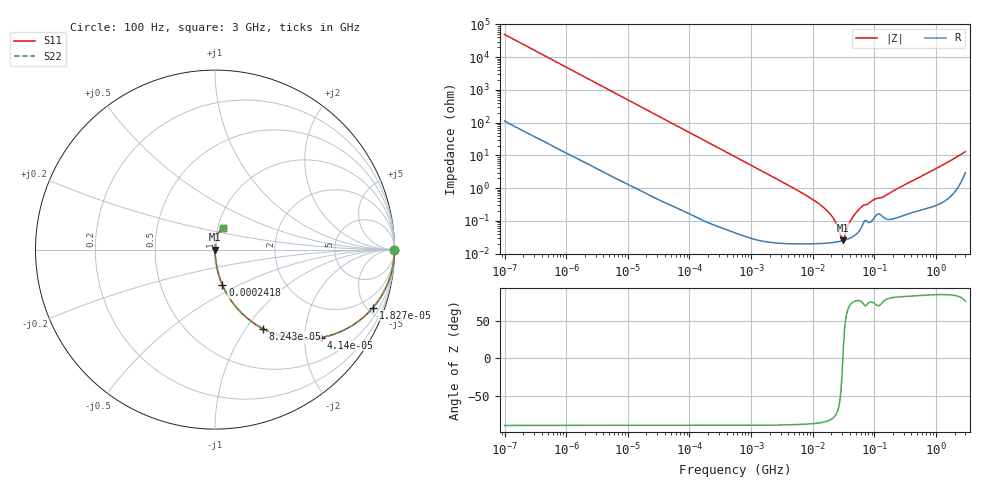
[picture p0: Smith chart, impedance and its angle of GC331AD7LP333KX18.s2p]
!Murata Part Number: GC331AD7LP333KX18
!These Parameters are Measured in Series Mode Connection
!Data Generated on Jun 10, 2025
!  o--ll--o
!Port1  Port2
!  o------o
!Operation Temp=25[degC], DC Bias Voltage=0[V]
!Freq. Start=100[Hz] Stop=3[GHz] 401[Steps]
# Hz S RI R 50
!Freq.(Hz) S11(Real) S11(Imag) S21(Real) S21(Imag) S12(Real) S12(Imag) S22(Real) S22(Imag)
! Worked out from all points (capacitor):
!   401 points, 100 Hz to 3 GHz, reference 50 ohm
!   read as one part in series: C = 32.2 nF near 109 Hz
!   lowest |Z| = 25.9 mohm at 31.31 MHz (marker M1)
!   series resonance near 30.8 MHz, so ESL is about 830 pH
!   S11 on the Smith chart (normalised r, x): 100 Hz: open; 18.27 kHz: 1.01, -5.45; 41.4 kHz: 1.01, -2.41; 82.43 kHz: 1.00, -1.21; 241.8 kHz: 1.00, -0.41; 3 GHz: 1.06, +0.25
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100  1 -0.00202  8.7e-06 0.00202  8.7e-06 0.00202  1 -0.00202
1788  0.9986 -0.036  0.00139 0.036  0.00139 0.036  0.9986 -0.036
6504  0.9829 -0.1285  0.0171 0.1285  0.0171 0.1285  0.9829 -0.1285
18274  0.8807 -0.3228  0.1193 0.3228  0.1193 0.3228  0.8807 -0.3228
31977  0.7079 -0.4533  0.2921 0.4533  0.2921 0.4533  0.7079 -0.4533
41399  0.5917 -0.4901  0.4083 0.4901  0.4083 0.4901  0.5917 -0.4901
82428  0.2691 -0.4419  0.7309 0.4419  0.7309 0.4419  0.2691 -0.4419
138163  0.1166 -0.3192  0.8834 0.3192  0.8834 0.3192  0.1166 -0.3192
241767  0.0417 -0.1982  0.9583 0.1982  0.9583 0.1982  0.0417 -0.1982
547723  0.00872 -0.0906  0.9913 0.0906  0.9913 0.0906  0.00872 -0.0906
9794414  0.000221 -0.00461  0.9998 0.00461  0.9998 0.00461  0.000221 -0.00461
1.442825e7  0.000213 -0.00272  0.9998 0.00272  0.9998 0.00272  0.000213 -0.00272
1.950129e7  0.000218 -0.00155  0.9998 0.00155  0.9998 0.00155  0.000218 -0.00155
2.418395e7  0.000228 -0.0008  0.9998 0.0008  0.9998 0.0008  0.000228 -0.0008
2.872754e7  0.000243 -0.000228  0.9998 0.000228  0.9998 0.000228  0.000243 -0.000228
3.131008e7  0.000253 5.53e-05  0.9997 -5.53e-05  0.9997 -5.53e-05  0.000253 5.53e-05
4.231884e7  0.000314 0.00108  0.9997 -0.00108  0.9997 -0.00108  0.000314 0.00108
5.9714e7  0.000571 0.00246  0.9994 -0.00246  0.9994 -0.00246  0.000571 0.00246
1.000898e8  0.00128 0.00438  0.9987 -0.00438  0.9987 -0.00438  0.00128 0.00438
1.751444e8  0.00115 0.00693  0.9988 -0.00693  0.9988 -0.00693  0.00115 0.00693
9.797344e8  0.00439 0.0384  0.9956 -0.0384  0.9956 -0.0384  0.00439 0.0384
3e9  0.0435 0.1182  0.9565 -0.1182  0.9565 -0.1182  0.0435 0.1182
